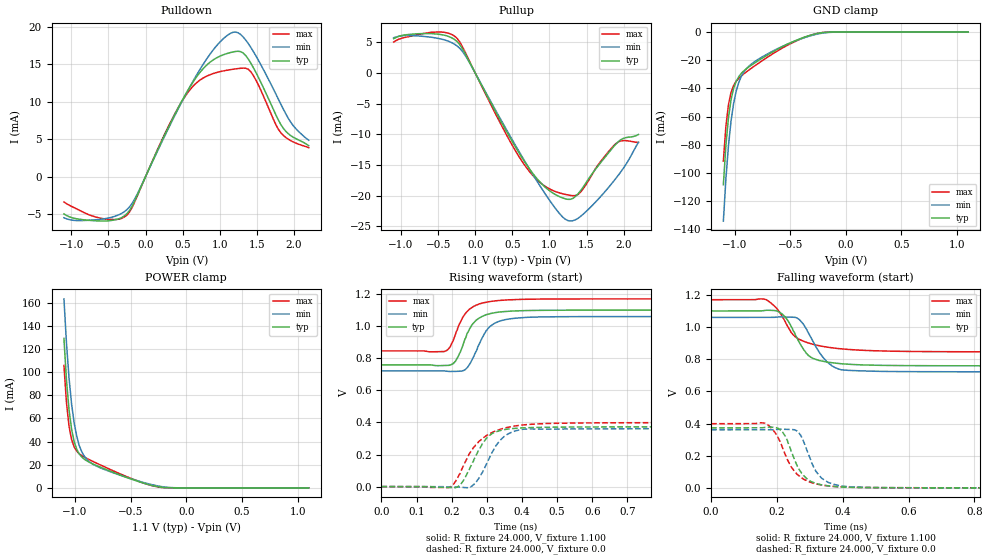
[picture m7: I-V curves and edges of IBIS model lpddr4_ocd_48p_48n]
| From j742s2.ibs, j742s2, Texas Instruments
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|   Model lpddr4_ocd_48p_48n
[Model] lpddr4_ocd_48p_48n
Model_type I/O
Polarity   Non-Inverting
Enable   Active-High
Vinl =  0.113V
Vinh =  0.253V
Vmeas =  0.183V
C_comp   1.679pF   1.501pF   1.938pF
[Model Spec]
Vinh   0.253V   0.247V   0.265V
Vinl   0.113V   0.107V   0.125V
Vmeas   0.183V   0.176V   0.195V
[Temperature Range]   25.000   0.125k   -40.000
[Voltage Range]   1.100V   1.060V   1.170V
[Pullup Reference]   1.100V   1.060V   1.170V
[Pulldown Reference]   0.0V   0.0V   0.0V
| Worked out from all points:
|   slope of the pulldown table from 0 to 0.165 V, typ, clamps not added: 45.8 ohm
|   slope of the pullup table from 0 to 0.165 V, typ, clamps not added: 43.3 ohm
|   GND clamp passes 1 mA (typ) near -0.25 V on its own axis
|   POWER clamp passes 1 mA (typ) near -0.26 V on its own axis
|   rising waveform, R_fixture 24.000, V_fixture 1.100: 20-80 % time 45.6ps typ, 48.5ps min, 45.8ps max; typ from 0.759 V to 1.1 V
|   rising waveform, R_fixture 24.000, V_fixture 0.0: 20-80 % time 55.3ps typ, 55.4ps min, 76.4ps max; typ from 0 V to 0.373 V
|   falling waveform, R_fixture 24.000, V_fixture 1.100: 20-80 % time 58.5ps typ, 61.7ps min, 79ps max; typ from 1.1 V to 0.759 V
|   falling waveform, R_fixture 24.000, V_fixture 0.0: 20-80 % time 51.3ps typ, 49.7ps min, 62.2ps max; typ from 0.373 V to 0 V
[Pulldown]
|Voltage   I(typ)   I(min)   I(max)
-1.1V     -4.95mA    -5.463mA   -3.355mA
-590mV    -5.893mA   -5.642mA   -5.544mA
-249mV    -4.895mA   -4.355mA   -5.082mA
295mV     6.337mA    6.167mA    6.44mA
567mV     11.46mA    11.43mA    11.19mA
839mV     15.01mA    15.91mA    13.47mA
1.179V    16.64mA    19.25mA    14.33mA
1.315V    16.5mA     18.64mA    14.48mA
1.418V    15.16mA    17.26mA    14.01mA
1.826V    6.924mA    9.641mA    5.845mA
1.996V    5.246mA    6.755mA    4.62mA
2.2V      4.144mA    4.87mA     3.879mA
[Pullup]
|Voltage   I(typ)   I(min)   I(max)
-1.1V     5.607mA    5.765mA    5.061mA
-590mV    6.441mA    5.844mA    6.657mA
-249mV    5.189mA    4.466mA    5.719mA
-113mV    2.652mA    2.453mA    2.832mA
397mV     -9.004mA   -8.724mA   -9.537mA
669mV     -14.55mA   -14.42mA   -15.09mA
941mV     -18.62mA   -19.69mA   -18.49mA
1.247V    -20.62mA   -24.08mA   -19.9mA
1.418V    -19.23mA   -23.43mA   -19.47mA
1.656V    -15.16mA   -20.62mA   -14.98mA
1.894V    -11.62mA   -17.23mA   -11.54mA
2.2V      -10.03mA   -11.3mA    -11.31mA
[GND_clamp]
|Voltage   I(typ)   I(min)   I(max)
-1.1V     -108.4mA   -134.2mA   -91.64mA
-1.077V   -80.17mA   -103.9mA   -66.63mA
-1.054V   -60.68mA   -80.47mA   -51.43mA
-1.031V   -48.01mA   -63.16mA   -42.83mA
-1.008V   -40.05mA   -50.75mA   -37.96mA
-985mV    -35.04mA   -42.04mA   -34.98mA
-940mV    -29.42mA   -31.64mA   -31.22mA
-894mV    -26.11mA   -26.16mA   -28.35mA
-848mV    -23.5mA    -22.73mA   -25.7mA
-527mV    -8.739mA   -8.686mA   -9.514mA
-229mV    -630.6uA   -1.042mA   -565.7uA
1.1V      0A         0A         0A
[POWER_clamp]
|Voltage   I(typ)   I(min)   I(max)
-1.1V     129.2mA    163.4mA    105.9mA
-1.077V   92.86mA    124.8mA    73.4mA
-1.054V   67.3mA     94.73mA    53.17mA
-1.031V   50.48mA    72.25mA    41.67mA
-1.008V   39.92mA    56.03mA    35.37mA
-985mV    33.38mA    44.6mA     31.76mA
-963mV    29.31mA    36.69mA    29.53mA
-917mV    24.75mA    27.38mA    26.61mA
-871mV    22.09mA    22.57mA    24.31mA
-619mV    11.98mA    11.76mA    13.12mA
-229mV    602.6uA    1.183mA    400.7uA
1.1V      0A         0A         0A
[Ramp]
| variable   typ   min   max
dV/dt_r   0.224/55.206p   0.217/54.962p   0.239/76.656p
dV/dt_f   0.205/57.871p   0.203/61.076p   0.195/76.757p
R_load = 24.000
[Rising Waveform]
R_fixture= 24.000
V_fixture= 1.100
V_fixture_min= 1.060
V_fixture_max= 1.170
|time   V(typ)   V(min)   V(max)
0s        758.8mV    721.5mV    845.8mV
181ps     754.7mV    720.3mV    843.3mV
197ps     758.3mV    717.4mV    876.5mV
210ps     778.8mV    718.3mV    945.3mV
234ps     895.9mV    723.8mV    1.065V
263ps     1.023V     813.2mV    1.124V
292ps     1.066V     949.6mV    1.146V
307ps     1.077V     994.9mV    1.153V
373ps     1.094V     1.048V     1.165V
3ns       1.1V       1.06V      1.17V
[Rising Waveform]
R_fixture= 24.000
V_fixture= 0.0
V_fixture_min= 0.0
V_fixture_max= 0.0
|time   V(typ)   V(min)   V(max)
0s        168.2uV    277.5uV    309.9uV
195ps     -5.512mV   -3.619mV   -3.108mV
223ps     8.947mV    -2.707mV   78.63mV
253ps     122.3mV    -2.849mV   214.7mV
281ps     243.8mV    65.03mV    288.1mV
314ps     330.7mV    210.2mV    336.2mV
334ps     347.6mV    278.4mV    354.4mV
357ps     357.8mV    324.9mV    369.1mV
429ps     368.4mV    359.1mV    389mV
3ns       373mV      361.2mV    399mV
[Falling Waveform]
R_fixture= 24.000
V_fixture= 1.100
V_fixture_min= 1.060
V_fixture_max= 1.170
|time   V(typ)   V(min)   V(max)
0s        1.1V       1.06V      1.17V
165ps     1.104V     1.06V      1.172V
215ps     1.083V     1.063V     1.07V
242ps     1.009V     1.062V     969.1mV
260ps     935.6mV    1.057V     933.1mV
295ps     823.6mV    966.2mV    901mV
350ps     783mV      786.7mV    875.8mV
385ps     773.7mV    739.6mV    866.5mV
425ps     767.7mV    729.8mV    859.5mV
3ns       758.8mV    721.5mV    845.8mV
[Falling Waveform]
R_fixture= 24.000
V_fixture= 0.0
V_fixture_min= 0.0
V_fixture_max= 0.0
|time   V(typ)   V(min)   V(max)
0s        373mV      361.2mV    399mV
166ps     377mV      361.2mV    400.5mV
198ps     374.4mV    362.9mV    332.9mV
217ps     347.7mV    364.6mV    248.4mV
242ps     236.3mV    363.3mV    134.3mV
256ps     163mV      359.5mV    96.47mV
281ps     75.94mV    287.5mV    53.72mV
323ps     25.07mV    88.96mV    22.56mV
380ps     7.576mV    17.9mV     7.599mV
3ns       168.2uV    277.1uV    309.8uV
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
